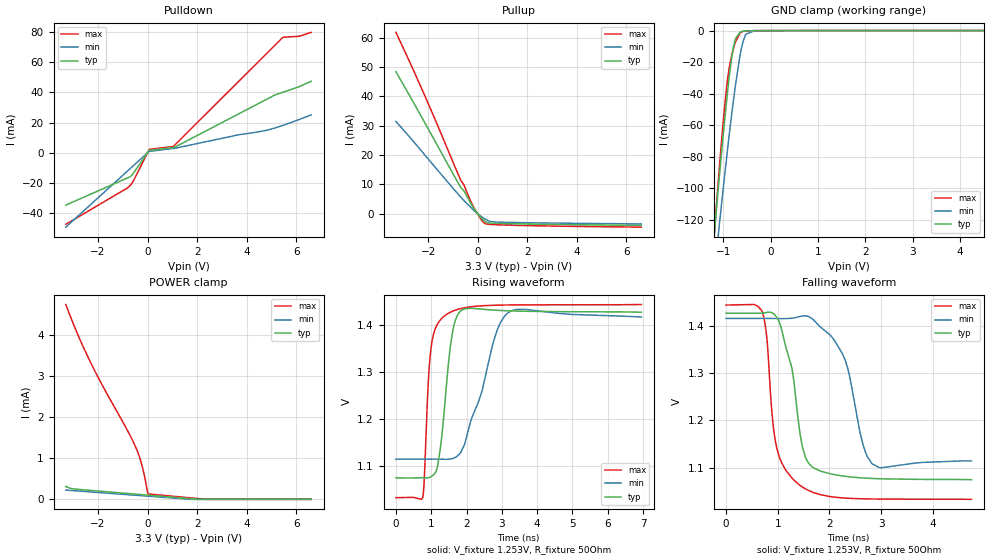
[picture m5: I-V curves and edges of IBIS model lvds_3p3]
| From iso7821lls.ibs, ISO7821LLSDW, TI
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|   lvds_3p3 Model
[Model]   lvds_3p3
Model_type   3-state
Polarity   Non-Inverting
Vmeas = 1.253
Vref = 1.253
Cref = 2pF
Rref = 50
|   typ   min   max
|   (nom PVT)   (fast PVT)   (slow PVT)
C_comp   4.329e-12   4.325e-12   5.375e-12
| Where nom  PVT is Nominal Process, 3.3V, 27C
|   Fast PVT is Strong Process,  3.6V, -55C
|   Slow PVT is Weak Process,   3V, 150C
[Voltage Range]   3.3   3   3.6
|Junction Temperature
[Temperature Range]   27   150   -55
[Pullup Reference]   3.3   3   3.6
[Pulldown Reference]   0   0   0
[Power Clamp Reference]   3.3   3   3.6
[GND Clamp Reference]   0   0   0
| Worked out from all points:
|   slope of the pulldown table from 0 to 0.495 V, typ, clamps not added: 209 ohm
|   slope of the pullup table from 0 to 0.495 V, typ, clamps not added: 159 ohm
|   GND clamp passes 1 mA (typ) near -0.64 V on its own axis
|   falling waveform, V_fixture 1.253V, R_fixture 50Ohm: 20-80 % time 320ps typ, 419ps min, 257ps max; typ from 1.43 V to 1.07 V
|   rising waveform, V_fixture 1.253V, R_fixture 50Ohm: 20-80 % time 276ps typ, 690ps min, 188ps max; typ from 1.07 V to 1.43 V
[Pulldown]
|   Voltage   I(typ)   I(min)   I(max)
-3.3V     -34.65mA   -49.24mA   -47.36mA
-852mV    -16.9mA    -12.68mA   -23.72mA
-693.6mV  -15.76mA   -10.31mA   -21.5mA
-576mV    -13.52mA   -8.558mA   -18.62mA
66mV      1.619mA    970.4uA    2.287mA
1.033V    3.483mA    2.889mA    4.155mA
3.691V    25.96mA    12mA       47.62mA
4.709V    34.67mA    14.61mA    64.27mA
5.135V    38.31mA    16.45mA    71.23mA
5.459V    40.12mA    18.17mA    76.53mA
6.131V    43.94mA    22.2mA     77.25mA
6.6V      47.37mA    25.12mA    79.82mA
[GND Clamp]
|   Voltage   I(typ)   I(min)   I(max)
-3.3V     -969.4mA   -865.9mA   -1.11A
-1.198V   -131.7mA   -157mA     -132.5mA
-1.111V   -102mA     -131.5mA   -97.8mA
-1.075V   -90.03mA   -121mA     -84.08mA
-988.8mV  -62.37mA   -96.68mA   -53.7mA
-918mV    -41.35mA   -77.55mA   -32.82mA
-789mV    -11.17mA   -45.29mA   -11.95mA
-738mV    -5.02mA    -33.79mA   -6.962mA
-636mV    -945.3uA   -14.23mA   -1.455mA
-525mV    -176.4uA   -2.347mA   -201.8uA
-330mV    -79.54uA   -87.29uA   -88.68uA
6.6V      0A         0A         0A
[Pullup]
|   Voltage   I(typ)   I(min)   I(max)
-3.3V     48.41mA    31.46mA    61.84mA
-2.087V   30.28mA    19.57mA    39.3mA
-682.8mV  8.93mA     5.658mA    11.36mA
-557.7mV  7.782mA    4.492mA    9.885mA
-330mV    4.263mA    2.624mA    5.141mA
-142.8mV  1.646mA    1.024mA    1.876mA
118.8mV   -1.237mA   -793.8uA   -1.75mA
234mV     -2.219mA   -1.468mA   -2.98mA
408mV     -3.052mA   -2.295mA   -3.568mA
594mV     -3.206mA   -2.763mA   -3.684mA
858mV     -3.281mA   -2.882mA   -3.78mA
6.6V      -3.987mA   -3.487mA   -4.571mA
[POWER Clamp]
|   Voltage   I(typ)   I(min)   I(max)
-3.3V     314.8uA    225.2uA    4.747mA
-2.843V   244.6uA    204.8uA    4.053mA
-2.346V   219.4uA    182.5uA    3.392mA
-1.818V   193uA      158.9uA    2.77mA
-859.2mV  145.1uA    115.9uA    1.73mA
-489mV    126.6uA    99.38uA    1.281mA
-249mV    114.6uA    88.63uA    874.7uA
-135.3mV  108.9uA    83.53uA    595.4uA
-2.4mV    102.3uA    77.56uA    176uA
26.4mV    100.8uA    76.27uA    132.7uA
2.356V    0A         0A         0A
6.6V      0A         0A         0A
[Ramp]
R_load = 50
|   typ   min   max
dV/dt_r   0.108466/6.91523e-10  0.0944536/8.69655e-10   0.126715/5.83172e-10
dV/dt_f   0.211095/3.2053e-10   0.180676/4.17139e-10   0.246413/2.56922e-10
[Falling Waveform]
V_fixture = 1.253V
V_fixture_min = 1.267V
V_fixture_max = 1.241V
R_fixture = 50Ohm
|   Time   V(typ)   V(min)   V(max)
0s        1.427V     1.416V     1.444V
697ps     1.427V     1.416V     1.431V
792ps     1.429V     1.416V     1.372V
962.1ps   1.421V     1.415V     1.152V
1.272ns   1.312V     1.416V     1.079V
1.386ns   1.21V      1.419V     1.067V
1.598ns   1.11V      1.42V      1.052V
2.264ns   1.083V     1.338V     1.036V
2.821ns   1.077V     1.109V     1.034V
4.75ns    1.075V     1.115V     1.033V
[Rising Waveform]
V_fixture = 1.253V
V_fixture_min = 1.267V
V_fixture_max = 1.241V
R_fixture = 50Ohm
|   Time   V(typ)   V(min)   V(max)
0s        1.075V     1.115V     1.033V
758ps     1.075V     1.115V     1.033V
993.4ps   1.077V     1.115V     1.351V
1.174ns   1.098V     1.115V     1.402V
1.349ns   1.202V     1.115V     1.418V
1.541ns   1.354V     1.115V     1.427V
1.742ns   1.421V     1.122V     1.433V
2.854ns   1.431V     1.386V     1.442V
3.2ns     1.43V      1.427V     1.443V
6.95ns    1.427V     1.417V     1.444V
